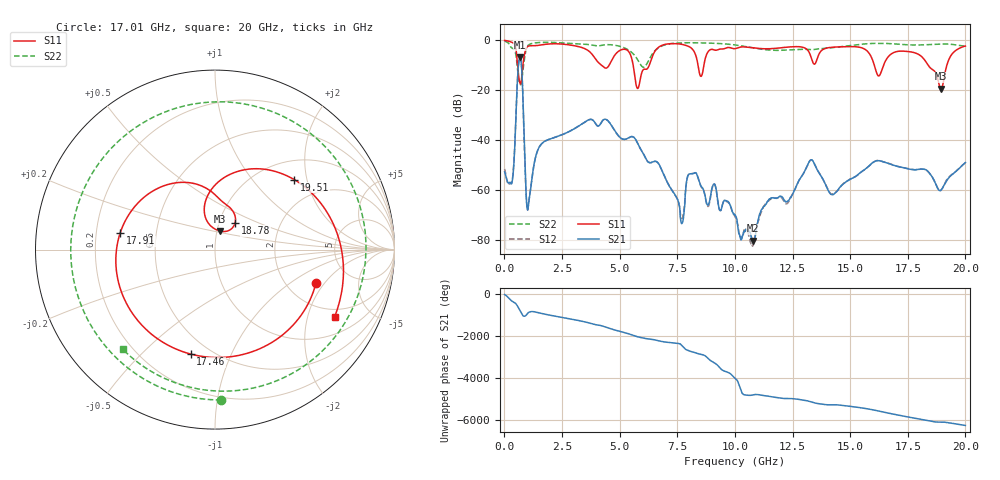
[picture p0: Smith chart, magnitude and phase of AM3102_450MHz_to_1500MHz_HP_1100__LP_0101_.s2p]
!Agilent Technologies,E8364B,MY43040894,A.07.50.67
!Agilent E8364B: A.07.50.67
!Date: Thursday, January 11, 2018 06:33:11
!Correction: S11(Full 2 Port(1,2))
!S21(Full 2 Port(1,2))
!S12(Full 2 Port(1,2))
!S22(Full 2 Port(1,2))
!S2P File: Measurements: S11, S21, S12, S22:
# Hz S  dB  R 50
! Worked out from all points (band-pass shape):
!   1601 points, 10 MHz to 20 GHz, reference 50 ohm
!   highest |S21| = -6.71 dB at 672.2 MHz (marker M1); lowest = -80.2 dB at 10.79 GHz (marker M2)
!   |S21| within 3 dB of the highest: 613 MHz to 738 MHz (125 MHz wide, 18.5 % of centre)
!   lowest |S11| = -19.4 dB at 18.94 GHz (marker M3), VSWR 1.24, Z = 51.8 + j10.8 ohm
!   |S11| at or under -10 dB: 5.587 GHz to 6.286 GHz (698.7 MHz wide, 11.8 % of centre); 16.05 GHz to 16.45 GHz (400.4 MHz wide, 2.46 % of centre); 18.38 GHz to 19.2 GHz (811 MHz wide, 4.32 % of centre)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
!   |S22| runs from -17.8 to -0.4 dB; largest |S21 - S12| = 0.011
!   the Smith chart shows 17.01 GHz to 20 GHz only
!   S11 on the Smith chart (normalised r, x): 17.01 GHz: 2.88, -1.64; 17.46 GHz: 0.39, -0.71; 17.91 GHz: 0.30, +0.08; 18.78 GHz: 1.19, +0.37; 19.51 GHz: 1.41, +1.68; 20 GHz: 1.66, -2.98
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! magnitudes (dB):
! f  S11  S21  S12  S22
! 10 MHz  -0.1  -52.7  -51.5  -0.4
! 334.8 MHz  -0.9  -56.8  -56.3  -3.2
! 672.2 MHz  -17.0  -6.7  -6.7  -17.6
! 1.034 GHz  -2.4  -66.8  -66.6  -2.0
! 1.559 GHz  -1.9  -42.1  -42.1  -0.9
! 3.346 GHz  -2.9  -33.6  -33.6  -1.5
! 5.782 GHz  -19.3  -41.3  -41.3  -7.8
! 6.682 GHz  -2.9  -49.3  -49.3  -3.0
! 7.706 GHz  -1.7  -73.3  -71.3  -1.0
! 8.218 GHz  -4.3  -53.2  -53.2  -1.0
! 10.01 GHz  -3.4  -69.8  -70.5  -1.9
! 10.79 GHz  -3.0  -80.2  -82.0  -3.0
! 13.34 GHz  -7.8  -47.9  -47.9  -3.8
! 14.23 GHz  -2.8  -61.8  -61.6  -3.0
! 16.68 GHz  -6.4  -49.3  -49.3  -1.3
! 17.01 GHz  -4.5  -50.4  -50.3  -1.5
! 17.46 GHz  -4.5  -51.4  -51.3  -1.8
! 17.91 GHz  -5.4  -51.7  -51.7  -1.9
! 18.78 GHz  -14.6  -58.9  -58.8  -1.6
! 18.94 GHz  -19.4  -60.1  -59.9  -1.5
! 19.51 GHz  -4.6  -53.1  -53.0  -1.8
! 20 GHz  -2.3  -48.9  -49.1  -2.4
